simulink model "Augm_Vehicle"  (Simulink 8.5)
settings: Solver=ode45  StartTime=0.0  StopTime=10.0  RelTol=1e-3
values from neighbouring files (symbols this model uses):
  wo = 0.0011    [start.m]    (also in start1.m; start2.m; start3.m)
undefined symbols (not defined in the file or in its folder): Al, Bl, Cl, Dl

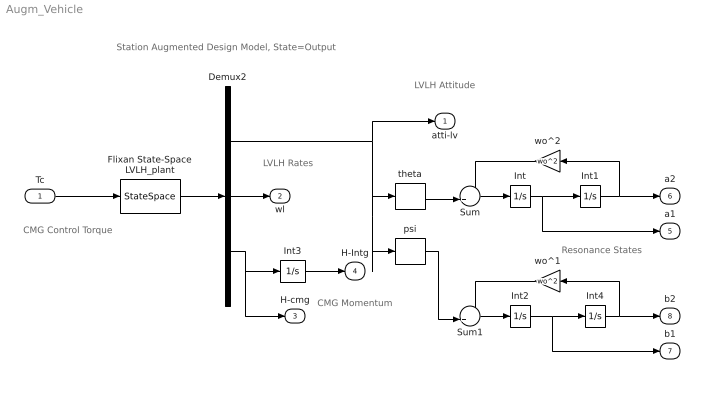
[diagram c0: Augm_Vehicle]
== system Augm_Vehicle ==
  note: LVLH Attitude
  note: LVLH Rates
  note: Resonance States
  note: CMG Control Torque
  note: CMG Momentum
  note: Station Augmented Design Model, State=Output
  Tc : Inport  PortDimensions=3
  Demux2 : Demux  Outputs=[3, 3, 3]
  Flixan State-Space LVLH_plant : StateSpace  A=Al  B=Bl  C=Cl  D=Dl  X0=0
  Int{,1..4} (5 alike) : Integrator
  Sum : Sum  Inputs=-+|
  Sum1 : Sum  Inputs=-+|
  psi : Selector  InputPortWidth=3  Indices=[3]
  theta : Selector  InputPortWidth=3  Indices=[2]
  wo^1 : Gain  Gain=wo^2
  wo^2 : Gain  Gain=wo^2
  atti-lv : Outport
  wl : Outport  Port=2
  H-cmg : Outport  Port=3
  H-Intg : Outport  Port=4
  a1 : Outport  Port=5
  a2 : Outport  Port=6
  b1 : Outport  Port=7
  b2 : Outport  Port=8
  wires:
  Demux2/1 -> psi/1, theta/1, atti-lv/1
  Int/1 -> Int1/1, a1/1
  Sum/1 -> Int/1
  Int1/1 -> a2/1, wo^2/1
  wo^2/1 -> Sum/1
  theta/1 -> Sum/2
  Flixan State-Space LVLH_plant/1 -> Demux2/1
  Demux2/2 -> wl/1
  Demux2/3 -> Int3/1, H-cmg/1
  Int3/1 -> H-Intg/1
  Tc/1 -> Flixan State-Space LVLH_plant/1
  Int2/1 -> Int4/1, b1/1
  Sum1/1 -> Int2/1
  Int4/1 -> b2/1, wo^1/1
  wo^1/1 -> Sum1/1
  psi/1 -> Sum1/2
